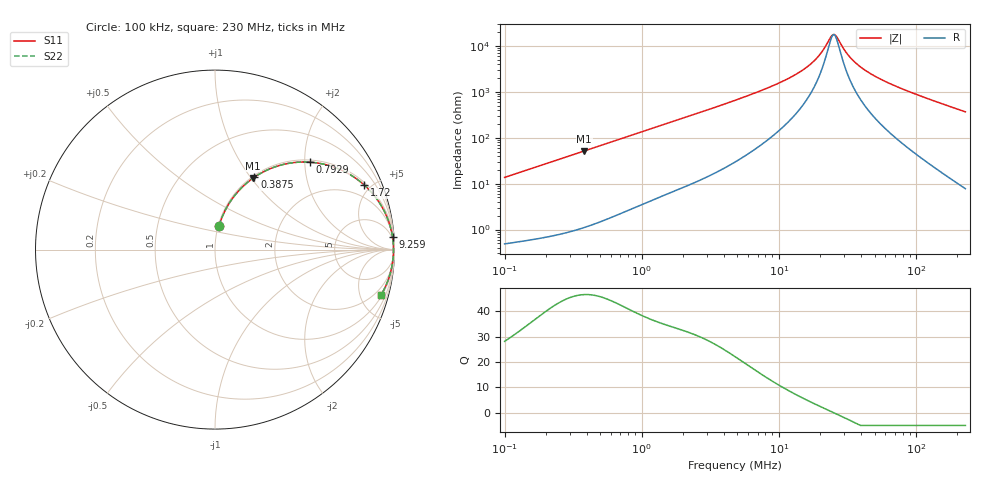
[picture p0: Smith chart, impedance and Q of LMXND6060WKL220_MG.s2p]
! LMXND6060WKL220_MG  S-PARAMETER MODEL  ( General Type )
! Model Generated by TAIYO YUDEN Corporation (https://www.yuden.co.jp/en/)
! Version 1.0
! TAIYO YUDEN Control No. 191025NI43SB-FBB
! Copyright(c) 2019 TAIYO YUDEN CO.,LTD. All Rights Reserved.
! Product Description (link to TY-COMPAS)
! https://ds.yuden.co.jp/TYCOMPAS/or/detail?pn=LMXND6060WKL220MMG&u=M
! Products Name : Inductors
! Characteristics :
!  Inductance : 22 uH , SRF(min) : 11 MHz , DC Resistance(max) : 0.348 Ohm
!  Rated Current : Saturation :1250 mA , Temp Rise : 950 mA (40 degC)
!  Case Size : 6.0 x 6.0 / 0.236 x 0.236 [mm/inch] , Thickness : 2 / 0.079 [mm/inch]
!  (Conditions: Temperature = 25 degC , DC Bias Current/Voltage = 0A / 0V)
! External Node Assignments :
!  1  o---GGG---o  2
! GND o---------o GND
! Frequency Range : 0.1MHz  -  229.966873MHz  [ 402 STEP ]
# MHz S RI R 50
! Freq[MHz].  S11 Real  S11 Imag  S21 Real  S21 Imag  S12 Real  S12 Imag  S22 Real  S22 Imag
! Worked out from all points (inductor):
!   401 points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, 100 kHz to 230 MHz, reference 50 ohm
!   read as one part in series: L = 21.7 uH near 103.9 kHz
!   highest Q = 46.6 at 380.1 kHz (marker M1), where L = 21.5 uH
!   self-resonance near 24.84 MHz
!   S11 on the Smith chart (normalised r, x): 100 kHz: 1.01, +0.27; 387.5 kHz: 1.02, +1.05; 792.9 kHz: 1.05, +2.13; 1.72 MHz: 1.14, +4.58; 9.259 MHz: 3, +28; 230 MHz: 1.16, -7.33
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0.1  0.0228 0.1327  0.9772 -0.1327  0.9772 -0.1327  0.0228 0.1327
0.208621  0.0794 0.2584  0.9206 -0.2584  0.9206 -0.2584  0.0794 0.2584
0.365661  0.2011 0.3902  0.7989 -0.3902  0.7989 -0.3902  0.2011 0.3902
0.380091  0.2134 0.3991  0.7866 -0.3991  0.7866 -0.3991  0.2134 0.3991
0.387518  0.2198 0.4035  0.7802 -0.4035  0.7802 -0.4035  0.2198 0.4035
0.792949  0.5304 0.487  0.4696 -0.487  0.4696 -0.487  0.5304 0.487
1.337081  0.7549 0.4163  0.2451 -0.4163  0.2451 -0.4163  0.7549 0.4163
1.719539  0.8326 0.3587  0.1674 -0.3587  0.1674 -0.3587  0.8326 0.3587
2.735974  0.9229 0.2504  0.0771 -0.2504  0.0771 -0.2504  0.9229 0.2504
4.889189  0.9717 0.1446  0.0283 -0.1446  0.0283 -0.1446  0.9717 0.1446
9.259215  0.9891 0.07  0.0109 -0.07  0.0109 -0.07  0.9891 0.07
13.37375  0.9926 0.0404  0.00735 -0.0404  0.00735 -0.0404  0.9926 0.0404
17.53523  0.9939 0.0222  0.00612 -0.0222  0.00612 -0.0222  0.9939 0.0222
20.47127  0.9942 0.0125  0.00576 -0.0125  0.00576 -0.0125  0.9942 0.0125
23.89891  0.9944 0.00319  0.00559 -0.00319  0.00559 -0.00319  0.9944 0.00319
25.3274  0.9944 -0.000283  0.00557 0.000283  0.00557 0.000283  0.9944 -0.000283
26.84128  0.9944 -0.00376  0.00558 0.00376  0.00558 0.00376  0.9944 -0.00376
31.94778  0.9942 -0.0143  0.00576 0.0143  0.00576 0.0143  0.9942 -0.0143
37.297  0.9939 -0.024  0.00613 0.024  0.00613 0.024  0.9939 -0.024
47.04613  0.9929 -0.0397  0.00713 0.0397  0.00713 0.0397  0.9929 -0.0397
64.11956  0.9903 -0.0641  0.00969 0.0641  0.00969 0.0641  0.9903 -0.0641
229.9669  0.9262 -0.2511  0.0738 0.2511  0.0738 0.2511  0.9262 -0.2511
